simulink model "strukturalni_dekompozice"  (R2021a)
settings: Solver=VariableStepAuto  StartTime=0.0  StopTime=10.0  RelTol=1e-3
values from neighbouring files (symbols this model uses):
  A = A(1:(pocet_stavu),1:(pocet_stavu))    [appDekompLQR.m]    (also in appLQR.m = A(1:(2*N-1),1:(2*N-1)); appSYM.m = A(1:(2*N-1),1:(2*N-1)); appSZV.m = A(1:(2*N-1),1:(2*N-1)); central_LQR.m = A(1:(2*N-1),1:(2*N-1)))
  a_lead = A(1,1)    [appDekompLQR.m]    (also in distri_STRUKTURAL.m; struktural_stary.m)
  ABk1 = a1 - b1*K_lead1    [struktural_stary.m]
  ABk2 = a2 - b2*K1    [struktural_stary.m]
  B = zeros(pocet_stavu,N)    [appDekompLQR.m]    (also in appLQR.m = zeros(2*N-1,N); appSYM.m = zeros(2*N-1,N); appSZV.m = zeros(2*N-1,N); central_LQR.m = zeros(2*N-1,N))
  B1 = B(1:3,2)    [struktural_stary.m]
  B2 = B(3:5,3)    [struktural_stary.m]
  b_lead = B(1,1)    [appDekompLQR.m]    (also in distri_STRUKTURAL.m; struktural_stary.m)
  C = eye(pocet_stavu)    [appDekompLQR.m]    (also in appLQR.m; appSYM.m; appSZV.m; central_LQR.m)
  D = zeros(pocet_stavu,N)    [appDekompLQR.m]    (also in appLQR.m; appSYM.m; appSZV.m; central_LQR.m)
  K = zeros(N,pocet_stavu)    [appDekompLQR.m]    (also in appSYM.m = [[0,-1/5,0,-3/20,0,-1/10,0,-1/20,0]; appSZV.m = [[-5/2,-3,7/4,1/2,0,0,0];[-1/7,-2/7,-7/2,-37/7,18/7,0,0];[0,; central_LQR.m = -K; central_SYM.m = [[0,-1/5,0,-3/20,0,-1/10,0,-1/20,0])
undefined symbols (not defined in the file or in its folder): K1, K2, K_lead, KKK
libraries: simulink x2

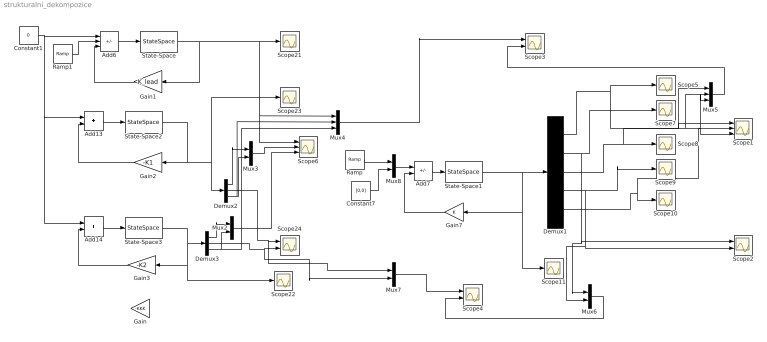
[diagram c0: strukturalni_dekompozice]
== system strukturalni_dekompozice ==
  Add13 : Sum
  Add14 : Sum
  Add6 : Sum  Inputs=++-
  Add7 : Sum  Inputs=+-
  Constant1 : Constant  Value=0
  Constant7 : Constant  Value=[0,0]
  Demux1 : Demux  Outputs=5
  Demux2 : Demux  Outputs=3
  Demux3 : Demux  Outputs=3
  Gain : Gain  Commented=on  Gain=-KKK  Multiplication=Matrix(K*u)
  Gain1 : Gain  Gain=K_lead
  Gain2 : Gain  Gain=-K1  Multiplication=Matrix(K*u)
  Gain3 : Gain  Gain=-K2  Multiplication=Matrix(K*u)
  Gain7 : Gain  Gain=K  Multiplication=Matrix(K*u)
  Mux{2..3,6..8} (5 alike) : Mux  Inputs=2
  Mux4 : Mux  Inputs=3
  Mux5 : Mux  Inputs=3
  Ramp : simulink/Sources/Ramp  slope=1  start=0  InitialOutput=0
  Ramp1 : simulink/Sources/Ramp  slope=1  start=0  InitialOutput=0
  Scope1 : Scope  NumInputPorts=3
  Scope{5,7..11,21..23} (9 alike) : Scope
  Scope{2..4,24} (4 alike) : Scope  NumInputPorts=2
  Scope6 : Scope  NumInputPorts=3
  State-Space : StateSpace  A=a_lead  B=b_lead  D=0  InitialCondition=1
  State-Space1 : StateSpace  A=A  B=B  C=C  D=D  InitialCondition=[0 1 0 0 0]
  State-Space2 : StateSpace  A=ABk1  B=B1  C=eye(3)  D=zeros(3,1)  InitialCondition=[0 0 0]
  State-Space3 : StateSpace  A=ABk2  B=B2  C=eye(3)  D=zeros(3,1)  InitialCondition=[0 0 0]
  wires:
  Mux2/1 -> Scope6/3
  Add13/1 -> State-Space2/1
  Gain3/1 -> Add14/2
  Demux3/1 -> Mux2/1
  Mux8/1 -> Add7/1
  Ramp/1 -> Mux8/1
  Demux1/5 -> Mux5/3, Scope1/3, Scope10/1
  Add14/1 -> State-Space3/1
  Mux7/1 -> Scope4/1
  Gain7/1 -> Add7/2
  Ramp1/1 -> Add6/2
  Constant7/1 -> Mux8/2
  Mux4/1 -> Scope3/1
  Mux6/1 -> Scope4/2
  State-Space2/1 -> Gain2/1, Scope23/1, Demux2/1
  Mux5/1 -> Scope3/2
  Demux3/3 -> Mux4/3, Mux2/2
  Demux1/1 -> Mux5/1, Scope1/1, Scope5/1
  Gain1/1 -> Add6/3
  Demux2/1 -> Mux3/1
  Mux3/1 -> Scope6/2
  State-Space1/1 -> Gain7/1, Scope11/1, Demux1/1
  Demux1/3 -> Mux5/2, Scope1/2, Scope8/1
  Add6/1 -> State-Space/1
  State-Space/1 -> Gain1/1, Mux4/1, Scope6/1, Scope21/1
  Demux1/4 -> Scope2/2, Mux6/2, Scope9/1
  State-Space3/1 -> Gain3/1, Scope22/1, Demux3/1
  Gain2/1 -> Add13/2
  Add7/1 -> State-Space1/1
  Demux2/2 -> Mux7/1, Scope24/1
  Demux1/2 -> Scope2/1, Mux6/1, Scope7/1
  Demux2/3 -> Mux4/2, Mux3/2
  Demux3/2 -> Mux7/2, Scope24/2
  Constant1/1 -> Add6/1, Add13/1, Add14/1
